(* Logix 5000 AddOnInstructionDefinition export AMCI_SD4840E2_Absolute_Move; software revision 20.03 *)

ADD_ON_INSTRUCTION AMCI_SD4840E2_Absolute_Move   (* revision 1.0, vendor AMCI, ExecuteEnableInFalse *)
VAR_INPUT
   Axis_Status_Bits : INT; {required}
   Type_0_for_standard_1_for_indexed : BOOL;
   Target_Position : DINT; {required}
   Programmed_Speed : DINT; {required}
   Acceleration : INT; {required}
   Deceleration : INT; {required}
   Jerk : INT;
END_VAR
VAR_IN_OUT
   AMCI_SD4840E2_output_data : _000A:SD4840E2_4342D302:O:0; {required}
END_VAR
VAR_OUTPUT
   EN : BOOL; {access Read Only, visible}
   ER : BOOL; {access Read Only, visible}
END_VAR
VAR
   Upper_Result_X_1000 : DINT;
   command_data_block : INT[10];
        [0]   // Command Bits MSW
        [1]   // Command Bits LSW
        [2]   // Upper Target Position
        [3]   // Lower Target Position
        [4]   // Upper Programmed Speed
        [5]   // Lower Programmed Speed
END_VAR

ROUTINE EnableInFalse   (* ladder *)
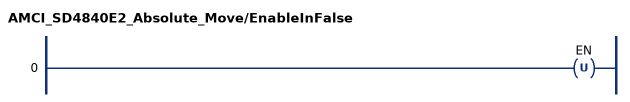
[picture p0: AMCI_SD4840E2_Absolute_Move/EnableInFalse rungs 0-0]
   0: OTU(EN);
END_ROUTINE

ROUTINE Logic   (* ladder *)
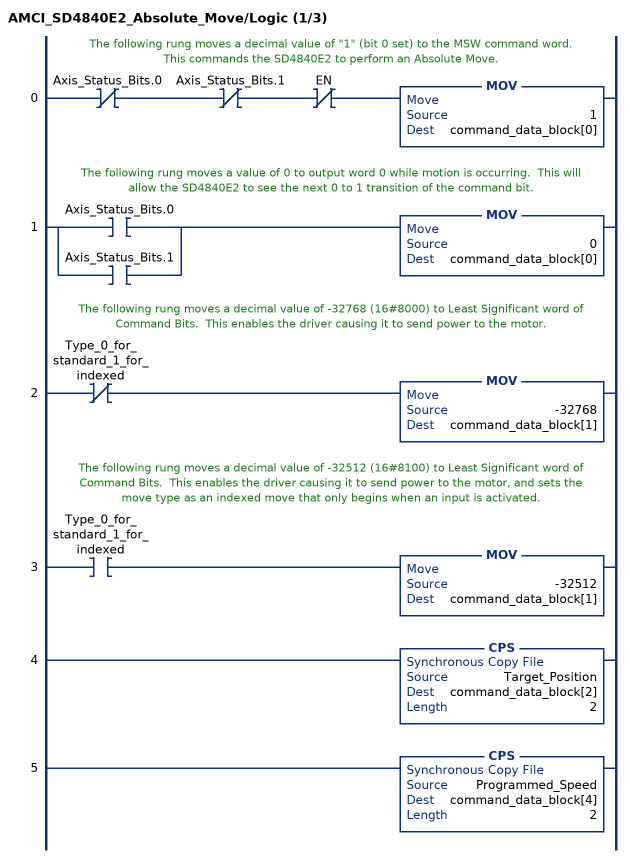
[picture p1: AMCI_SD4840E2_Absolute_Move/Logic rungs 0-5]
   // The following rung moves a decimal value of "1" (bit 0 set) to the MSW command word.  This commands the SD4840E2 to perform an Absolute Move.
   0: XIO(Axis_Status_Bits.0)XIO(Axis_Status_Bits.1)XIO(EN)MOV(1,command_data_block[0]);
   // The following rung moves a value of 0 to output word 0 while motion is occurring.  This will allow the SD4840E2 to see the next 0 to 1 transition of the command bit.
   1: [XIC(Axis_Status_Bits.0) ,XIC(Axis_Status_Bits.1) ]MOV(0,command_data_block[0]);
   // The following rung moves a decimal value of -32768 (16#8000) to Least Significant word of Command Bits.  This enables the driver causing it to send power to the motor.
   2: XIO(Type_0_for_standard_1_for_indexed)MOV(-32768,command_data_block[1]);
   // The following rung moves a decimal value of -32512 (16#8100) to Least Significant word of Command Bits.  This enables the driver causing it to send power to the motor, and sets the move type as an indexed move that only begins when an input is activated.
   3: XIC(Type_0_for_standard_1_for_indexed)MOV(-32512,command_data_block[1]);
   4: CPS(Target_Position,command_data_block[2],2);
   5: CPS(Programmed_Speed,command_data_block[4],2);
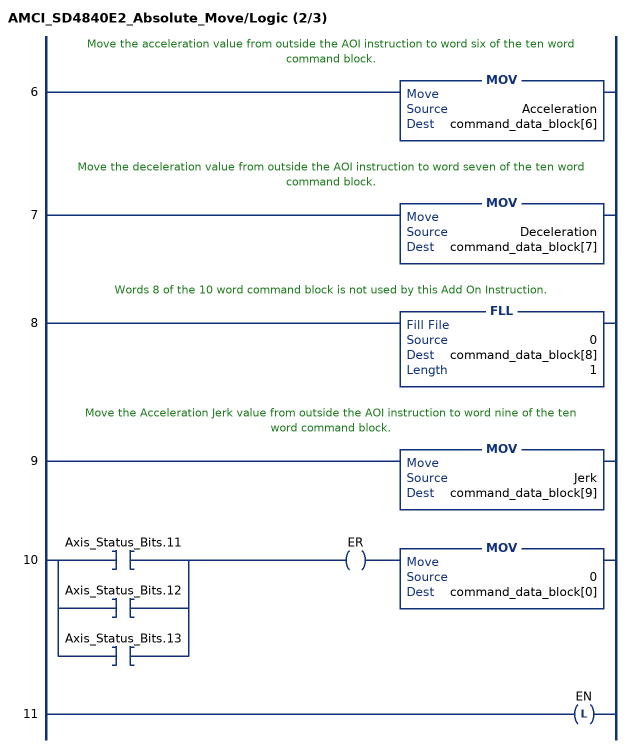
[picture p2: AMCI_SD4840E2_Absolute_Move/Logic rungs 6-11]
   // Move the acceleration value from outside the AOI instruction to word six of the ten word command block.
   6: MOV(Acceleration,command_data_block[6]);
   // Move the deceleration value from outside the AOI instruction to word seven of the ten word command block.
   7: MOV(Deceleration,command_data_block[7]);
   // Words 8 of the 10 word command block is not used by this Add On Instruction.
   8: FLL(0,command_data_block[8],1);
   // Move the Acceleration Jerk value from outside the AOI instruction to word nine of the ten word command block.
   9: MOV(Jerk,command_data_block[9]);
   10: [XIC(Axis_Status_Bits.11) ,XIC(Axis_Status_Bits.12) ,XIC(Axis_Status_Bits.13) ]OTE(ER)MOV(0,command_data_block[0]);
   11: OTL(EN);
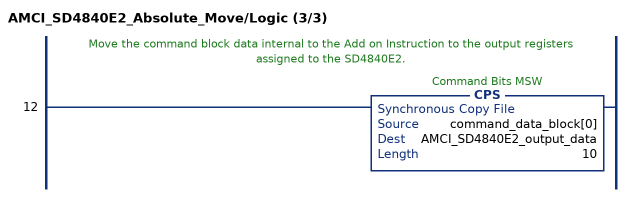
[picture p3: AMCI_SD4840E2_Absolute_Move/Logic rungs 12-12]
   // Move the command block data internal to the Add on Instruction to the output registers assigned to the SD4840E2.
   12: CPS(command_data_block[0],AMCI_SD4840E2_output_data,10);
END_ROUTINE
END_ADD_ON_INSTRUCTION
